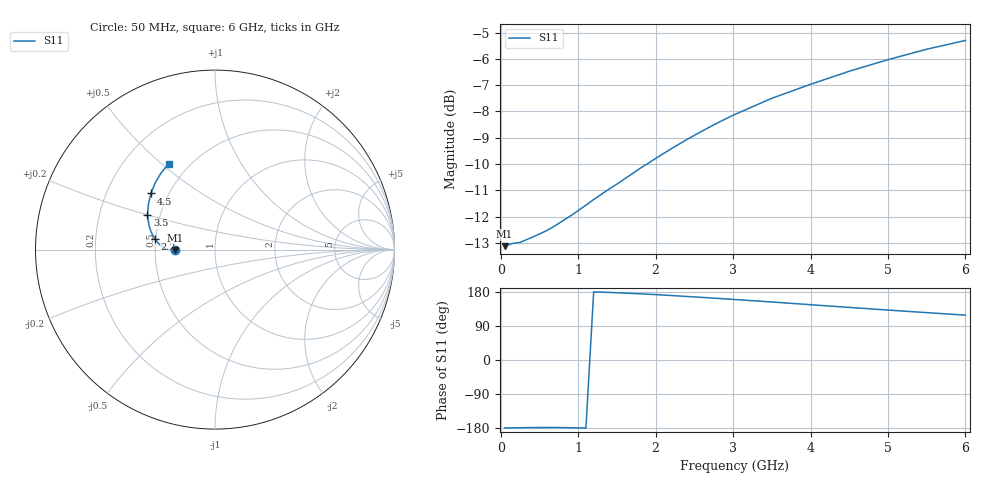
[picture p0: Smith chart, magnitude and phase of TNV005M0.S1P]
! SIEMENS Discrete & RF Semiconductors
! BAS70-07W
! Si Schottky Diode in SOT343
! IF = 5 mA
! S-Parameters:  February  1997
# GHz  S  MA  R  50
!  f  S11
! GHz  MAG  ANG
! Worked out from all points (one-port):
!   34 points, 50 MHz to 6 GHz, reference 50 ohm
!   lowest |S11| = -13.1 dB at 50 MHz (marker M1), VSWR 1.57, Z = 31.9 - j0.155 ohm
!   |S11| at or under -10 dB: start of sweep to 1.887 GHz
!   S11 on the Smith chart (normalised r, x): 50 MHz: 0.64, -0.00; 2.2 GHz: 0.50, +0.06; 3.5 GHz: 0.43, +0.20; 4.5 GHz: 0.40, +0.32; 6 GHz: 0.39, +0.53
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0.05  0.2209 -179.4
0.1  0.2223 -179.3
0.15  0.2234 -179.0
0.25  0.2245 -178.7
0.4  0.2295 -178.3
0.5  0.2329 -178.2
0.6  0.2367 -178.2
0.7  0.2414 -178.1
0.8  0.2467 -178.4
1  0.258 -179.1
1.1  0.2643 -179.6
1.3  0.2772 179.2
1.4  0.2836 178.4
1.5  0.2897 177.5
1.6  0.2965 176.6
1.8  0.3105 174.7
2  0.3242 172.6
2.2  0.3382 170.2
2.4  0.3519 167.7
2.6  0.3654 165.2
2.8  0.3787 162.6
3  0.3916 159.9
3.5  0.4217 153.1
4  0.4484 145.9
4.5  0.4747 138.8
5  0.4994 131.8
5.5  0.5227 125.0
6  0.5432 118.4
